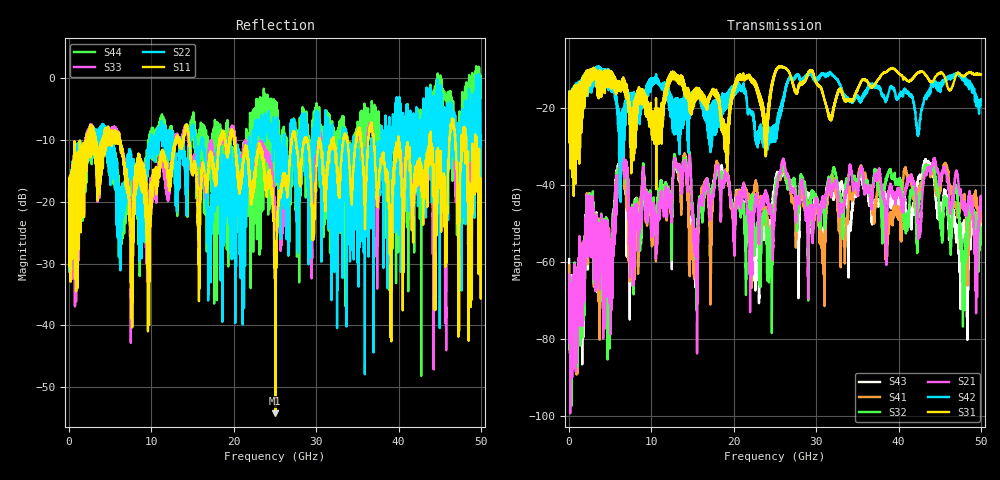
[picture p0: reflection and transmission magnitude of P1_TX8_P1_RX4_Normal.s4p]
!Keysight Technologies,N5225B,MY57041031,A.13.20.10
!Date: Friday, May 31, 2019 11:19:34
!Correction: S11(Full 4 Port(1,2,3,4))
!S12(Full 4 Port(1,2,3,4))
!S13(Full 4 Port(1,2,3,4))
!S14(Full 4 Port(1,2,3,4))
!S21(Full 4 Port(1,2,3,4))
!S22(Full 4 Port(1,2,3,4))
!S23(Full 4 Port(1,2,3,4))
!S24(Full 4 Port(1,2,3,4))
!S31(Full 4 Port(1,2,3,4))
!S32(Full 4 Port(1,2,3,4))
!S33(Full 4 Port(1,2,3,4))
!S34(Full 4 Port(1,2,3,4))
!S41(Full 4 Port(1,2,3,4))
!S42(Full 4 Port(1,2,3,4))
!S43(Full 4 Port(1,2,3,4))
!S44(Full 4 Port(1,2,3,4))
!S4P File: Measurements: <S11,S12,S13,S14>,
!<S21,S22,S23,S24>,
!<S31,S32,S33,S34>,
!<S41,S42,S43,S44>:
# Hz S  dB  R 50.0
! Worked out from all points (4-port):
!   5000 points, 10 MHz to 50 GHz, reference 50 ohm
!   strongest paths, dB at 10 MHz, 12.51 GHz, 25.01 GHz, 37.51 GHz, 50 GHz:
!     S31: -19.6, -10.8, -11.0, -12.6, -11.2
!     S42: -19.3, -19.3, -26.0, -14.8, -17.7
!     S21: -64.3, -42.8, -46.1, -36.9, -42.9
!     S32: -65.3, -46.7, -42.2, -40.3, -53.4
!     S41: -60.9, -42.8, -43.0, -39.0, -46.7
!     S43: -59.3, -46.8, -39.8, -44.6, -48.2
!   lowest |S11| = -54.2 dB at 25.05 GHz (marker M1), VSWR 1.00, Z = 49.8 - j0.0247 ohm
!   |S11| at or under -10 dB: 6.192 GHz to 12.89 GHz (6.696 GHz wide, 70.2 % of centre); 20.1 GHz to 26.99 GHz (6.893 GHz wide, 29.3 % of centre); 40 GHz to 43.77 GHz (3.765 GHz wide, 8.99 % of centre)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
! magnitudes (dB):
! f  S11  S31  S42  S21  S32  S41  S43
! 10 MHz  -19.5  -19.6  -19.3  -64.3  -65.3  -60.9  -59.3
! 5.06 GHz  -8.5  -10.9  -11.0  -67.8  -64.6  -63.2  -61.5
! 6.41 GHz  -11.9  -14.9  -33.8  -31.1  -30.2  -30.3  -29.7
! 14.06 GHz  -8.5  -15.5  -22.7  -34.9  -34.2  -32.6  -32.6
! 15.33 GHz  -14.3  -15.8  -16.9  -55.8  -56.3  -56.7  -62.1
! 25.05 GHz  -54.2  -10.5  -24.8  -44.6  -42.0  -41.4  -39.5
! 50 GHz  -22.7  -11.2  -17.7  -42.9  -53.4  -46.7  -48.2
